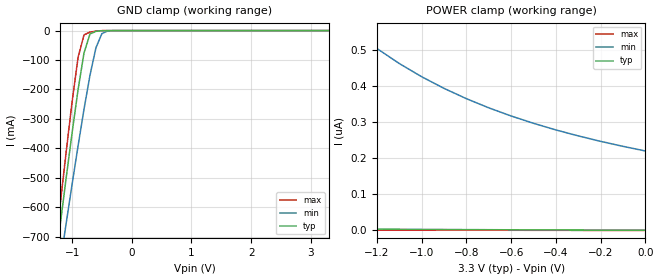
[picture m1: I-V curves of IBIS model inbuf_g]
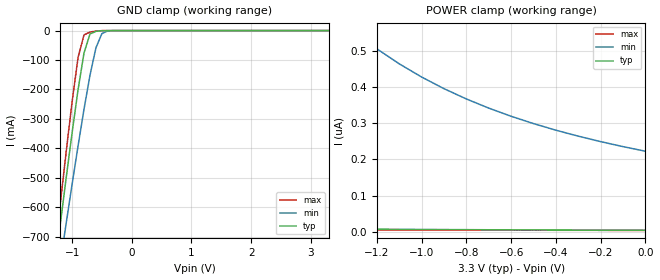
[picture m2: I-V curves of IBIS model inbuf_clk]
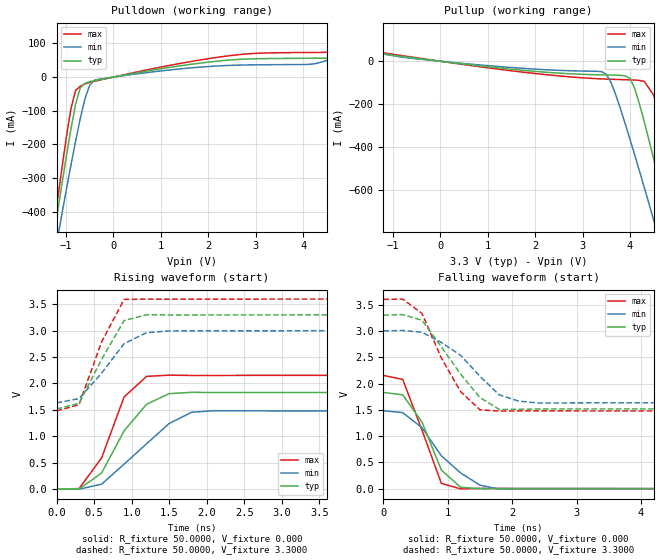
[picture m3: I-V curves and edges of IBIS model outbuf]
| IBIS file 5v2310z_tssop_3p3.ibs created by s2ibis2 version 1.2
| North Carolina State University Electronics Research Laboratory  1995
[IBIS ver]   2.1
[File name]   5v2310z.ibs
[File Rev]   0.4
[Date]   02/26/2004 jbp
[Source]   Integrated Device Technology, Inc.
[Notes]   1.Temperatures: typ=25C, min=150C, max=-40C 2.RRmp rates based
   on 500 ohm load and 25pF.
[Disclaimer] Integrated Device Technology, Inc. ("IDT") hereby grants the
   user of this IBIS model a non-exclusive, nontransferable
   license to use this IBIS model under the following terms. The
   user is granted this license only to use the IBIS model and is
   not granted rights to sell, copy (except as needed to run the
   IBIS model), rent, lease or sub-license the IBIS model in
   whole or in part, or in modified form to anyone. The User may
   modify the IBIS model to suit its specific applications, but
   rights to derivative works and such modifications shall belong
   to IDT. This IBIS model is provided on an AS IS" basis and IDT
   makes absolutely no warranty with respect to the information
   contained herein. IDT DISCLAIMS AND CUSTOMER WAIVES ALL
   WARRANTIES, EXPRESS AND IMPLIED, INCLUDING WARRANTIES OF
   MERCHANTABILITY AND FITNESS FOR A PARTICULAR PURPOSE. THE
   ENTIRE RISK AS TO QUALITY AND PERFORMANCE IS WITH THE USER
   ACCORDINGLY, IN NO EVENT SHALL IDT BE LIABLE FOR ANY DIRECT OR
   INDIRECT DAMAGES, WHETHER IN CONTRACT OR TORT, INCLUDING ANY
   LOST PROFITS OR OTHER INCIDENTAL, CONSEQUENTIAL, EXEMPLARY, OR
   PUNITIVE DAMAGES ARISING OUT OF THE USE OR APPLICATION OF THE
   IBIS model. Further, IDT reserves the right to make changes
   without notice to any product herein to improve reliability,
   function, or design. IDT does not convey any license under
   patent rights or any other intellectual property rights,
   including those of third parties. IDT is not obligated to
   provide maintenance or support for the licensed IBIS model.
[Copyright]   Copyright 1997, Integrated Device Technology, Inc. all rights
   reserved
|   Component idt5v2310z
[Component]   idt5v2310z
[Manufacturer]   Integrated Device Technology, Inc.
[Package]
| variable   typ   min   max
R_pkg   91.60m   81.80m   101.4m
L_pkg   3.14nH   2.64nH   3.65nH
C_pkg   0.390pF   0.314pf   0.462pF
[Pin]  signal_name   model_name   R_pin   L_pin   C_pin
1   GND   GND
2   VDD   POWER
3   Y10   outbuf
4   Y11   outbuf
5   Y12   outbuf
6   GND   GND
7   GND   GND
8   Y13   outbuf
9   Y14   outbuf
10   VDD   POWER
11   G1   inbuf_g
12   Y24   outbuf
13   G2   inbuf_g
14   VDD   POWER
15   VDD   POWER
16   Y23   outbuf
17   Y22   outbuf
18   GND   GND
19   GND   GND
20   Y21   outbuf
21   Y20   outbuf
22   VDD   POWER
23   VDD   POWER
24   CLK   inbuf_clk
| Models and submodels in the file (3): inbuf_g (Input), inbuf_clk (Input), outbuf (Output)
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|   Model inbuf_g
[Model]   inbuf_g
Model_type   Input
Polarity   Non-Inverting
Vinl =   0.8000V
Vinh =   2.0000V
C_comp   3.0000pF   NA   NA
[Temperature Range]   25.0000   0.1500k   -40.0000
[Voltage Range]   3.3000V   3.0000V   3.6000V
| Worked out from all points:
|   GND clamp passes 1 mA (typ) near -0.52 V on its own axis
[GND_clamp]
| voltage   I(typ)   I(min)   I(max)
-3.3V     -4.178A    -3.771A    -4.57A
-1.3V     -823mA     -929.4mA   -775.2mA
-1.2V     -661.4mA   -792.1mA   -592.7mA
-1.1V     -502.3mA   -656.3mA   -413.9mA
-1V       -347.6mA   -522.7mA   -242.5mA
-900mV    -201.2mA   -392.2mA   -91.4mA
-800mV    -75.82mA   -267mA     -14.55mA
-700mV    -11.63mA   -151.7mA   -5.267mA
-600mV    -2.491mA   -58.09mA   -1.497mA
-500mV    -519.6uA   -10.16mA   -175.5uA
-400mV    -56.6uA    -1.033mA   -10.24uA
3.3V      713.1pA    261.4nA    -296.8pA
[POWER_clamp]
| voltage   I(typ)   I(min)   I(max)
-3.3V     51.34nA    5.138uA    3.942nA
-2.9V     30.56nA    3.218uA    3.247nA
-2.5V     18.22nA    2.007uA    2.684nA
-2V       9.699nA    1.128uA    2.082nA
-1.3V     4.236nA    550.2nA    1.327nA
-1.2V     3.78nA     503nA      1.223nA
-1.1V     3.374nA    461.5nA    1.12nA
-1V       3.01nA     425nA      1.017nA
-800mV    2.389nA    364.3nA    812.6pA
-600mV    1.874nA    316.4nA    609.5pA
-400mV    1.436nA    277.9nA    407.3pA
0V        713.1pA    219.7nA    4.512pA
|   Model inbuf_clk
[Model]   inbuf_clk
Model_type   Input
Polarity   Non-Inverting
Vinl =   0.8000V
Vinh =   2.0000V
C_comp   3.0000pF   NA   NA
[Temperature Range]   25.0000   0.1500k   -40.0000
[Voltage Range]   3.3000V   3.0000V   3.6000V
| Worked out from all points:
|   GND clamp passes 1 mA (typ) near -0.52 V on its own axis
[GND_clamp]
| voltage   I(typ)   I(min)   I(max)
-3.3V     -4.178A    -3.771A    -4.57A
-1.3V     -823mA     -929.4mA   -775.2mA
-1.2V     -661.4mA   -792.1mA   -592.7mA
-1.1V     -502.3mA   -656.3mA   -413.9mA
-1V       -347.6mA   -522.7mA   -242.5mA
-900mV    -201.2mA   -392.2mA   -91.4mA
-800mV    -75.82mA   -267mA     -14.55mA
-700mV    -11.63mA   -151.7mA   -5.267mA
-600mV    -2.491mA   -58.09mA   -1.497mA
-500mV    -519.6uA   -10.16mA   -175.5uA
-400mV    -56.6uA    -1.033mA   -10.24uA
3.3V      4.013nA    264.4nA    3.303nA
[POWER_clamp]
| voltage   I(typ)   I(min)   I(max)
-3.3V     54.64nA    5.141uA    7.542nA
-2.9V     33.86nA    3.221uA    6.847nA
-2.5V     21.52nA    2.01uA     6.284nA
-1.4V     8.05nA     607nA      5.031nA
-1.3V     7.536nA    553.2nA    4.927nA
-1.2V     7.08nA     506nA      4.823nA
-1.1V     6.674nA    464.5nA    4.72nA
-1V       6.31nA     428nA      4.617nA
-800mV    5.689nA    367.3nA    4.413nA
-600mV    5.174nA    319.4nA    4.21nA
-400mV    4.736nA    280.9nA    4.007nA
0V        4.013nA    222.7nA    3.605nA
|   Model outbuf
[Model]   outbuf
Model_type   Output
Polarity   Non-Inverting
Vmeas =   1.6500V
Cref =  25.0000pF
Rref =   0.5000k
C_comp   3.0000pF   NA   NA
[Temperature Range]   25.0000   0.1500k   -40.0000
[Voltage Range]   3.3000V   3.0000V   3.6000V
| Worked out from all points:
|   slope of the pulldown table from 0 to 0.495 V, typ, clamps not added: 38.9 ohm
|   slope of the pullup table from 0 to 0.495 V, typ, clamps not added: 37.4 ohm
|   rising waveform, R_fixture 50.0000, V_fixture 0.000: 20-80 % time 491ps typ, 695ps min, 376ps max; typ from 0 V to 1.83 V
|   rising waveform, R_fixture 50.0000, V_fixture 3.3000: 20-80 % time 409ps typ, 465ps min, 368ps max; typ from 1.52 V to 3.3 V
|   falling waveform, R_fixture 50.0000, V_fixture 0.000: 20-80 % time 411ps typ, 630ps min, 392ps max; typ from 1.83 V to 0 V
|   falling waveform, R_fixture 50.0000, V_fixture 3.3000: 20-80 % time 651ps typ, 728ps min, 518ps max; typ from 3.3 V to 1.52 V
[Pulldown]
| voltage   I(typ)   I(min)   I(max)
-3.3V     -2.435A    -2.209A    -2.656A
-1.3V     -510.7mA   -574.6mA   -486.5mA
-1V       -241.5mA   -340.2mA   -185.5mA
-900mV    -157.6mA   -264.8mA   -96.88mA
-800mV    -82.13mA   -192.1mA   -40.11mA
-700mV    -31.94mA   -123.8mA   -27.05mA
-600mV    -18.49mA   -64.19mA   -20.2mA
-300mV    -7.94mA    -6.197mA   -9.372mA
2.4V      50.05mA    34.48mA    62.72mA
4.2V      56.06mA    38.74mA    73.26mA
5.5V      82.95mA    93.56mA    74.58mA
6.6V      141.6mA    144.4mA    134.2mA
[Pullup]
| voltage   I(typ)   I(min)   I(max)
-3.3V     139.8mA    129.1mA    149.7mA
-700mV    19.57mA    16.13mA    22.72mA
3.4V      -63.66mA   -48.72mA   -82.36mA
3.6V      -64.58mA   -99.66mA   -84.17mA
4V        -79.62mA   -364.9mA   -86.87mA
4.3V      -282.4mA   -588.1mA   -93.82mA
4.5V      -455mA     -742.1mA   -158.5mA
4.7V      -632.9mA   -901.7mA   -339.3mA
4.9V      -813.2mA   -1.063A    -537.6mA
5.1V      -995.3mA   -1.226A    -740.6mA
5.3V      -1.182A    -1.389A    -945.7mA
6.6V      -2.441A    -2.461A    -2.333A
[Ramp]
| variable   typ   min   max
dV/dt_r   1.8438/0.4131n   1.6482/0.5659n   2.0322/0.3172n
dV/dt_f   1.8395/0.5169n   1.6337/0.6423n   2.0296/0.4069n
R_load = 0.5000k
[Rising Waveform]
R_fixture = 50.0000
V_fixture = 0.000
| time   V(typ)   V(min)   V(max)
0s        -238.8uV   -150.7uV   -341.8uV
300ps     -599.5uV   -2.394mV   8.156mV
600ps     303.3mV    92.3mV     589.1mV
900ps     1.103V     472.5mV    1.746V
1.2ns     1.607V     858.5mV    2.135V
1.5ns     1.808V     1.242V     2.158V
1.8ns     1.833V     1.456V     2.152V
2.1ns     1.829V     1.484V     2.153V
15ns      1.83V      1.482V     2.154V
[Rising Waveform]
R_fixture = 50.0000
V_fixture = 3.3000
V_fixture_min = 3.0000
V_fixture_max = 3.6000
| time   V(typ)   V(min)   V(max)
0s        1.516V     1.633V     1.478V
300ps     1.624V     1.714V     1.601V
600ps     2.456V     2.196V     2.788V
900ps     3.193V     2.756V     3.594V
1.2ns     3.303V     2.964V     3.598V
1.5ns     3.299V     2.995V     3.597V
15ns      3.3V       3V         3.6V
[Falling Waveform]
R_fixture = 50.0000
V_fixture = 0.000
| time   V(typ)   V(min)   V(max)
0s        1.83V      1.482V     2.154V
300ps     1.785V     1.446V     2.078V
600ps     1.266V     1.159V     1.111V
900ps     353.5mV    625.4mV    100mV
1.2ns     26.01mV    298.4mV    -4.932mV
1.5ns     -884.7uV   66.33mV    3.171mV
1.8ns     2.807mV    -10.21mV   2.26mV
2.4ns     1.286mV    1.52mV     831.7uV
15ns      0V         1.541uV    0V
[Falling Waveform]
R_fixture = 50.0000
V_fixture = 3.3000
V_fixture_min = 3.0000
V_fixture_max = 3.6000
| time   V(typ)   V(min)   V(max)
0s        3.3V       3V         3.6V
300ps     3.31V      3.009V     3.607V
600ps     3.203V     2.975V     3.332V
900ps     2.698V     2.781V     2.486V
1.2ns     2.178V     2.536V     1.845V
1.5ns     1.732V     2.138V     1.5V
1.8ns     1.506V     1.782V     1.475V
2.1ns     1.509V     1.667V     1.479V
2.4ns     1.516V     1.629V     1.479V
15ns      1.516V     1.633V     1.478V
